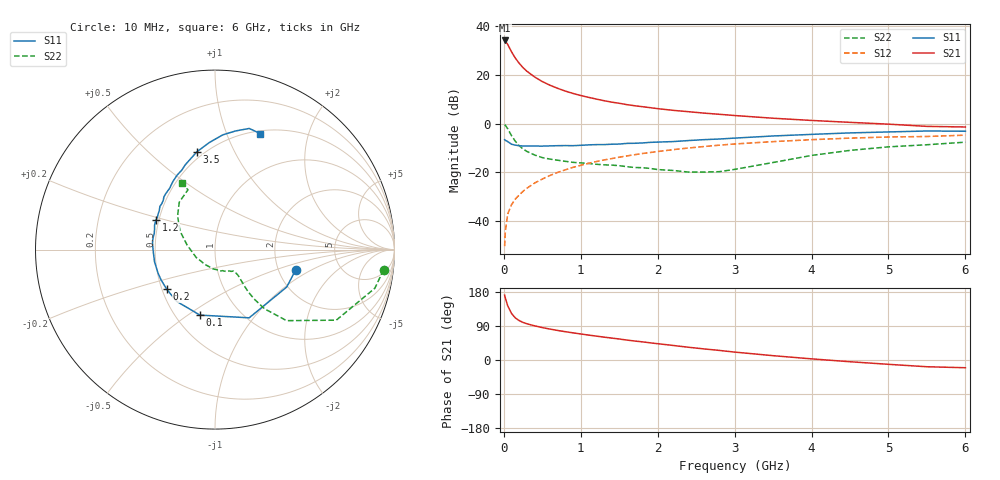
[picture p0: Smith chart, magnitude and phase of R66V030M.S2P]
! SIEMENS Small Signal Semiconductors
! BFR193
! Si NPN RF Bipolar Junction Transistor in SOT23
! VCE = 6 V  IC = 30 mA
! Common Emitter S-Parameters:  May  1996
# GHz  S  MA  R  50
!  f  S11  S21  S12  S22
! GHz  MAG  ANG  MAG  ANG  MAG  ANG  MAG  ANG
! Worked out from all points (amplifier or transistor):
!   36 points, 10 MHz to 6 GHz, reference 50 ohm
!   highest |S21| = 34.2 dB at 10 MHz (marker M1)
!   |S21| within 3 dB of that: start of sweep to 72.67 MHz
!   unconditionally stable (mu >= 1): 484.1 MHz to 2.021 GHz
!   at 250 MHz: K = 0.89, MSG = 25.4 dB, |S12| = -27.9 dB
!   at 1.4 GHz: K = 1.02, MAG = 10.7 dB, |S12| = -14.4 dB
!   at 6 GHz: K = 0.94, MSG = 1.7 dB, |S12| = -4.8 dB
!   lowest NFmin = 1.90 dB at 450 MHz
!   S11 on the Smith chart (normalised r, x): 10 MHz: 2.49, -0.72; 100 MHz: 0.66, -0.56; 200 MHz: 0.53, -0.27; 1.2 GHz: 0.48, +0.18; 3.5 GHz: 0.46, +0.72; 6 GHz: 0.53, +1.32
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0.01  0.4638 -14.1  51.07 171.3  0.003 85.4  0.9465 -6.8
0.02  0.4506 -27.6  49.43 163.2  0.0061 80.2  0.9162 -13.6
0.05  0.4251 -63.4  42.36 143.1  0.0137 70.0  0.7817 -30.2
0.1  0.3745 -103.0  29.87 122.7  0.0214 64.1  0.5617 -44.8
0.15  0.3589 -126.5  22.05 110.9  0.028 65.1  0.4297 -50.1
0.2  0.3483 -140.5  17.31 104.0  0.034 67.0  0.35 -51.6
0.25  0.3446 -150.3  14.06 99.1  0.0403 67.9  0.2984 -51.8
0.3  0.3434 -157.2  11.88 95.5  0.0467 69.5  0.2664 -51.2
0.4  0.3437 -168.4  9.073 90.2  0.0596 70.8  0.2249 -49.7
0.5  0.343 -175.0  7.287 85.5  0.0721 71.4  0.1989 -48.4
0.6  0.3462 178.6  6.123 81.6  0.0855 71.1  0.1853 -48.0
0.7  0.3502 173.7  5.287 77.9  0.0987 70.8  0.1757 -48.3
0.8  0.3514 169.7  4.641 74.7  0.1117 69.8  0.1667 -48.9
1.1  0.3636 157.8  3.455 65.8  0.1514 67.1  0.1509 -53.6
1.2  0.368 153.4  3.185 63.1  0.1645 65.9  0.1452 -55.4
1.6  0.39 141.9  2.443 52.6  0.2154 60.7  0.1293 -67.4
2.2  0.4249 126.5  1.866 38.4  0.2898 52.2  0.1082 -95.5
2.8  0.4797 112.7  1.548 25.3  0.3583 43.3  0.1022 -143.0
3.5  0.5541 100.5  1.284 11.4  0.4242 32.5  0.1578 170.6
4.5  0.6408 86.1  1.056 -4.6  0.5006 18.4  0.2801 138.1
5.5  0.7015 74.2  0.873 -17.8  0.5408 4.6  0.3658 114.3
6  0.6934 68.6  0.848 -20.4  0.576 0.5  0.4131 116.4
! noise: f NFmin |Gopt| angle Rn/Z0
0.45  1.9  0.4  180  0.09
0.9  1.95  0.43  -173  0.11
1.8  2.4  0.58  -144  0.24
